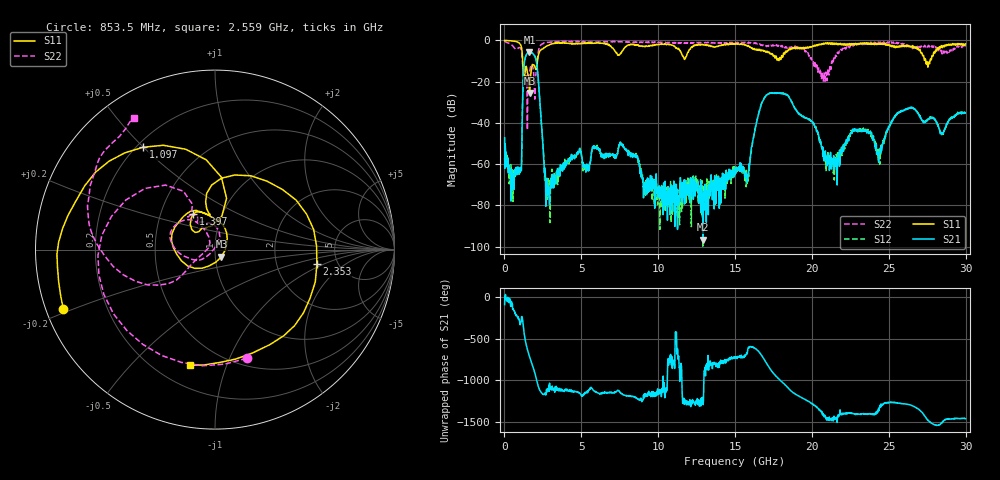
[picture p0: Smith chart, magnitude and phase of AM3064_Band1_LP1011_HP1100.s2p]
# Hz S DB R 50.0
!freq dBS11 angS11 dBS21 angS21 dBS12 angS12 dBS22 angS22
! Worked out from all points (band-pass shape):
!   1600 points, 10 MHz to 29.98 GHz, reference 50 ohm
!   highest |S21| = -5.65 dB at 1.622 GHz (marker M1); lowest = -96.6 dB at 12.92 GHz (marker M2)
!   |S21| within 3 dB of the highest: 1.344 GHz to 2.026 GHz (681.9 MHz wide, 40.5 % of centre)
!   lowest |S11| = -25.5 dB at 1.641 GHz (marker M3), VSWR 1.11, Z = 53.6 - j4.22 ohm
!   |S11| at or under -10 dB: 1.187 GHz to 2.147 GHz (960.4 MHz wide, 57.6 % of centre); 27.4 GHz to 27.68 GHz (282.1 MHz wide, 1.02 % of centre)
!   |S22| runs from -43.4 to -0.3 dB; largest |S21 - S12| = 0.0076
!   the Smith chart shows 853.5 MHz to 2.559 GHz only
!   S11 on the Smith chart (normalised r, x): 853.5 MHz: 0.05, -0.19; 1.097 GHz: 0.22, +0.50; 1.397 GHz: 0.73, +0.30; 2.353 GHz: 3.46, -0.85; 2.559 GHz: 0.33, -0.75
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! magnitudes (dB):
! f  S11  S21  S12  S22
! 10 MHz  -0.1  -47.2  -57.0  -0.3
! 853.5 MHz  -0.8  -63.8  -64.2  -4.0
! 1.097 GHz  -3.1  -63.2  -63.0  -4.9
! 1.397 GHz  -12.7  -7.4  -7.4  -16.5
! 1.622 GHz  -25.1  -5.7  -5.6  -15.6
! 1.641 GHz  -25.5  -5.7  -5.6  -14.8
! 2.053 GHz  -14.2  -9.4  -9.4  -15.5
! 2.353 GHz  -4.8  -35.1  -34.9  -2.3
! 2.559 GHz  -3.6  -58.5  -57.5  -1.3
! 2.84 GHz  -2.5  -71.3  -68.2  -1.0
! 5.015 GHz  -1.5  -56.2  -56.1  -0.7
! 7.601 GHz  -6.0  -49.9  -50.1  -0.7
! 10 GHz  -2.0  -72.6  -75.5  -1.0
! 12.92 GHz  -2.1  -96.6  -71.3  -1.1
! 15 GHz  -1.9  -65.2  -61.3  -1.4
! 15.79 GHz  -2.8  -68.4  -69.9  -1.3
! 17.14 GHz  -5.8  -26.0  -25.9  -2.8
! 19.99 GHz  -3.3  -39.2  -39.5  -9.3
! 21.36 GHz  -1.3  -59.0  -60.5  -11.4
! 22.67 GHz  -1.7  -42.9  -44.2  -2.7
! 25 GHz  -2.0  -42.3  -42.0  -1.0
! 29.98 GHz  -1.7  -35.1  -35.4  -3.0
